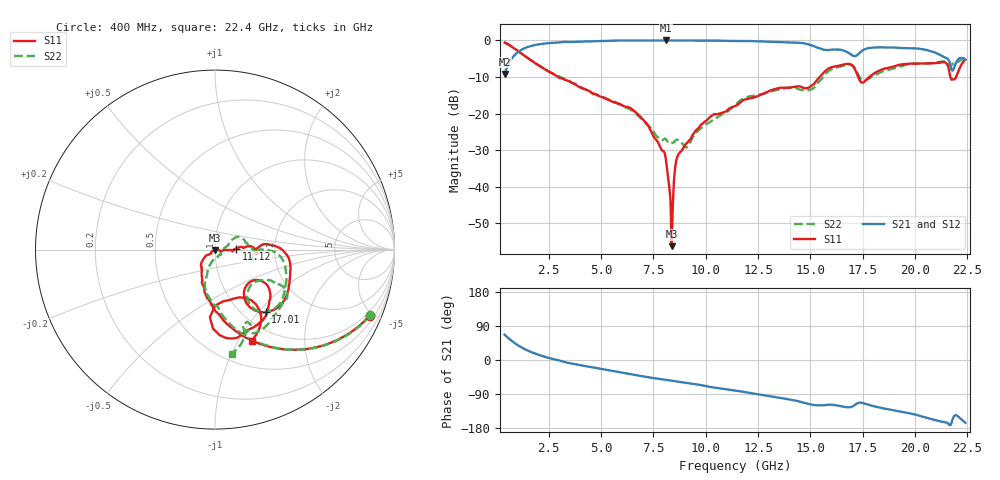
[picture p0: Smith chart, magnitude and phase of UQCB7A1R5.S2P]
!  Part Number  UQCB7A1R5	Mounting Orientation: Vertical
!  Description: RF capacitors
!  Application: Coupling, Bypass, Tuning, DC Block
!  Filters, Matching
# GHZ S DB R 50
! Freq  |S11|  S11 Ph  |S21|  S21 Ph  |S12|  S12 Ph  |S22|  S22 Ph
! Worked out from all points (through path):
!   401 points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, 400 MHz to 22.4 GHz, reference 50 ohm
!   highest |S21| = 0.00 dB at 8.1 GHz (marker M1); lowest = -9.2 dB at 400 MHz (marker M2)
!   group delay of S21, straight-line fit = 24.4 ps
!   lowest |S11| = -56.3 dB at 8.375 GHz (marker M3), VSWR 1.00, Z = 49.9 - j0.144 ohm
!   |S11| at or under -10 dB: 2.953 GHz to 15.44 GHz (12.49 GHz wide, 136 % of centre); 17.28 GHz to 17.81 GHz (531.2 MHz wide, 3.03 % of centre); 21.68 GHz to 21.96 GHz (275.5 MHz wide, 1.26 % of centre)
!   |S22| runs from -29.3 to -0.5 dB; largest |S21 - S12| = 0.0049
!   S11 on the Smith chart (normalised r, x): 400 MHz: 0.79, -4.76; 11.12 GHz: 1.27, +0.01; 17.01 GHz: 1.25, -1.10; 22.4 GHz: 0.79, -1.14
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0.4  -0.57 -23.1  -9.19 66.9  -9.18 66.8  -0.54 -23.0
0.95  -2.54 -48.1  -3.59 41.9  -3.58 41.9  -2.50 -47.8
1.83  -6.09 -72.9  -1.28 17.6  -1.26 17.5  -6.08 -71.8
4.085  -13.05 -105.5  -0.30 -14.2  -0.29 -14.3  -12.88 -103.6
6.505  -18.91 -133.2  -0.01 -38.3  -0.01 -38.5  -19.25 -109.1
7.77  -28.47 -140.0  -0.01 -49.8  -0.01 -50.0  -26.65 -85.0
8.1  -32.55 -147.4  0.00 -52.5  -0.02 -52.8  -26.94 -69.8
8.375  -56.27 -110.3  -0.01 -54.6  -0.03 -54.9  -28.02 -52.8
8.595  -32.78 -6.3  -0.02 -56.5  -0.04 -56.7  -27.14 -42.5
8.76  -30.70 -16.1  -0.02 -57.8  -0.04 -58.0  -27.36 -41.1
9.145  -27.82 -9.7  -0.01 -60.6  -0.01 -60.9  -28.93 -10.5
11.125  -18.61 2.2  -0.12 -78.5  -0.13 -78.7  -19.11 29.7
11.4  -17.98 3.2  -0.15 -80.7  -0.17 -80.8  -17.78 30.5
15.085  -12.24 3.3  -1.40 -118.0  -1.41 -118.0  -13.25 -4.8
16.02  -7.30 -13.0  -2.52 -118.1  -2.52 -118.2  -7.87 -14.0
17.01  -6.96 -51.0  -4.10 -122.7  -4.12 -122.7  -6.81 -48.8
17.505  -11.55 -43.7  -2.69 -113.6  -2.71 -113.6  -10.95 -46.9
18.77  -7.41 -45.0  -1.91 -130.6  -1.93 -130.5  -7.99 -28.5
20.695  -6.30 -69.4  -2.85 -154.8  -2.87 -154.7  -6.20 -44.6
21.41  -5.97 -80.1  -4.62 -163.9  -4.64 -163.9  -5.74 -62.2
21.795  -10.68 -73.7  -8.27 -155.5  -8.28 -155.7  -6.33 -66.1
22.4  -5.24 -68.1  -5.29 -165.9  -5.30 -165.9  -4.63 -80.9
